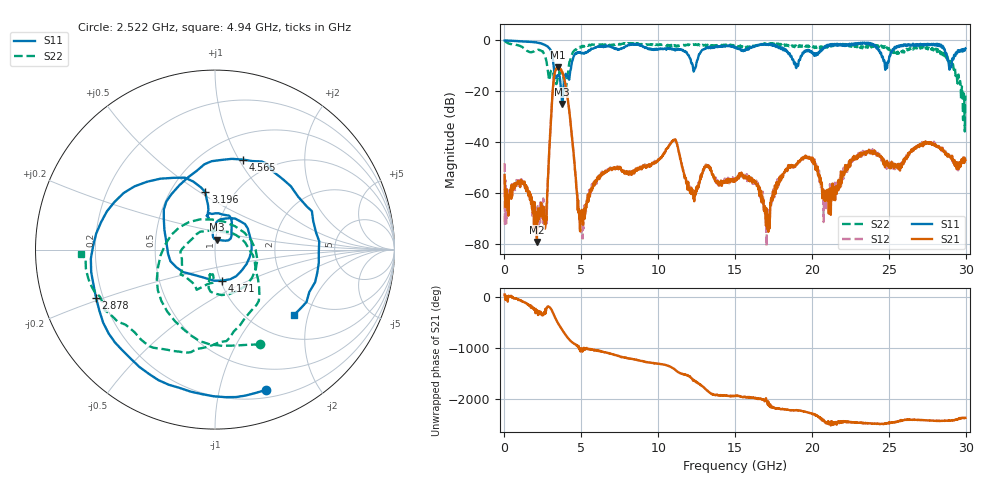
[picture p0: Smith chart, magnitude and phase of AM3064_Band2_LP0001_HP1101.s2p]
# Hz S DB R 50.0
!freq dBS11 angS11 dBS21 angS21 dBS12 angS12 dBS22 angS22
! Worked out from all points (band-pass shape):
!   1600 points, 10 MHz to 29.98 GHz, reference 50 ohm
!   highest |S21| = -10.67 dB at 3.496 GHz (marker M1); lowest = -79.2 dB at 2.109 GHz (marker M2)
!   |S21| within 3 dB of the highest: 3.245 GHz to 3.825 GHz (580.1 MHz wide, 16.4 % of centre)
!   lowest |S11| = -25.0 dB at 3.759 GHz (marker M3), VSWR 1.12, Z = 50.9 + j5.58 ohm
!   |S11| at or under -10 dB: 3.201 GHz to 4.349 GHz (1.148 GHz wide, 30.4 % of centre); 12.24 GHz to 12.46 GHz (215.3 MHz wide, 1.74 % of centre); 28.92 GHz to 29.08 GHz (163.3 MHz wide, 0.563 % of centre)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
!   |S22| runs from -35.8 to -0.2 dB; largest |S21 - S12| = 0.0074
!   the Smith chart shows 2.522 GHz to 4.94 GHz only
!   S11 on the Smith chart (normalised r, x): 2.522 GHz: 0.27, -1.40; 2.878 GHz: 0.17, -0.19; 3.196 GHz: 0.74, +0.53; 4.171 GHz: 1.02, -0.36; 4.565 GHz: 0.75, +1.04; 4.94 GHz: 1.50, -1.63
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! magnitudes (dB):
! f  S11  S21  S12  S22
! 10 MHz  -0.1  -52.9  -48.3  -0.2
! 2.109 GHz  -0.9  -79.2  -75.1  -3.9
! 2.522 GHz  -1.6  -67.2  -62.1  -4.7
! 2.878 GHz  -2.9  -48.8  -48.2  -14.5
! 3.196 GHz  -9.7  -15.8  -15.8  -14.2
! 3.496 GHz  -13.9  -10.7  -10.6  -14.5
! 3.759 GHz  -25.0  -12.4  -12.5  -14.0
! 4.171 GHz  -15.0  -25.5  -25.5  -10.7
! 4.565 GHz  -5.6  -48.7  -48.9  -3.8
! 4.94 GHz  -4.9  -67.7  -72.8  -2.5
! 5.015 GHz  -5.1  -68.7  -75.9  -2.7
! 6.327 GHz  -2.5  -52.8  -52.5  -1.6
! 10 GHz  -3.4  -46.8  -47.0  -1.7
! 12.25 GHz  -10.2  -60.4  -59.4  -1.7
! 15 GHz  -2.7  -54.3  -55.8  -1.9
! 17.09 GHz  -1.7  -67.8  -69.0  -1.6
! 19.99 GHz  -4.5  -47.2  -46.9  -2.2
! 21.15 GHz  -1.7  -63.5  -60.8  -2.0
! 23.14 GHz  -1.1  -45.1  -45.6  -3.0
! 25 GHz  -8.2  -49.7  -48.9  -3.0
! 28.56 GHz  -3.1  -43.4  -43.5  -4.9
! 29.98 GHz  -3.2  -47.0  -46.3  -21.7
